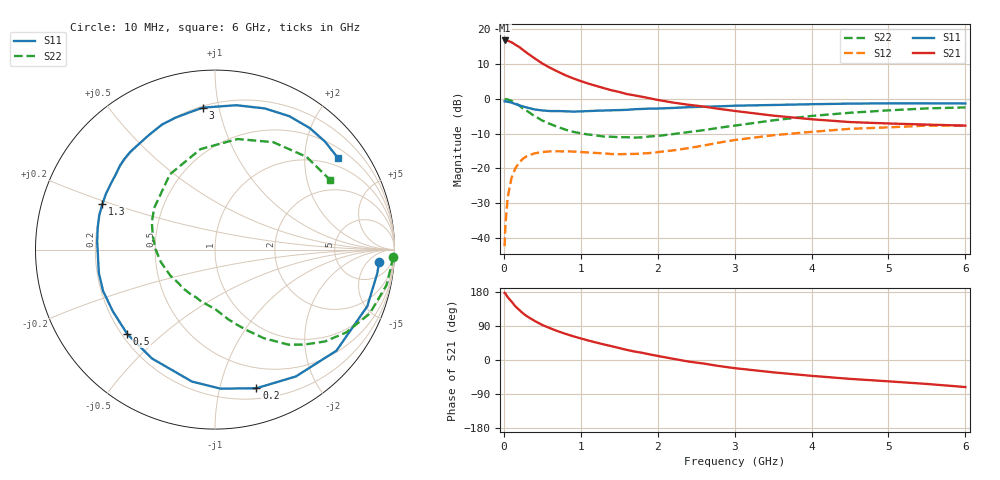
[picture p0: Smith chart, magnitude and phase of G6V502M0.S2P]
! SIEMENS Small Signal Semiconductors
! BFG193
! Si NPN RF Bipolar Junction Transistor in SOT223
! VCE = 0.5 V  IC = 2 mA
! Common Emitter S-Parameters:  August  1996
# GHz  S  MA  R  50
!  f  S11  S21  S12  S22
! GHz  MAG  ANG  MAG  ANG  MAG  ANG  MAG  ANG
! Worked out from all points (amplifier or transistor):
!   36 points, 10 MHz to 6 GHz, reference 50 ohm
!   highest |S21| = 16.8 dB at 10 MHz (marker M1)
!   |S21| within 3 dB of that: start of sweep to 265.8 MHz
!   unconditionally stable (mu >= 1): 1.313 GHz to end of sweep
!   at 250 MHz: K = 0.20, MSG = 15.6 dB, |S12| = -17.2 dB
!   at 1.4 GHz: K = 1.07, MAG = 7.5 dB, |S12| = -15.9 dB
!   at 6 GHz: K = 1.04, MAG = -1.2 dB, |S12| = -7.7 dB
!   S11 on the Smith chart (normalised r, x): 10 MHz: 13, -11; 200 MHz: 0.29, -1.30; 500 MHz: 0.22, -0.39; 1.3 GHz: 0.20, +0.19; 3 GHz: 0.21, +0.90; 6 GHz: 0.75, +2.84
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0.01  0.9175 -4.2  6.882 177.1  0.0076 88.4  0.9938 -2.4
0.02  0.9136 -8.4  6.88 175.4  0.0151 88.6  0.9874 -4.7
0.05  0.9055 -20.4  6.823 165.8  0.0381 78.0  0.976 -11.7
0.1  0.8803 -39.8  6.481 154.3  0.0727 68.4  0.9325 -22.5
0.15  0.8382 -57.5  5.98 141.6  0.1001 57.3  0.8652 -32.2
0.2  0.806 -73.4  5.537 132.2  0.1215 49.7  0.7981 -39.9
0.25  0.7755 -87.7  5.025 123.0  0.1377 42.4  0.7243 -47.0
0.3  0.7464 -99.9  4.557 115.5  0.15 36.8  0.6683 -52.4
0.4  0.7009 -120.1  3.812 103.2  0.1642 28.2  0.5627 -61.2
0.5  0.6784 -136.1  3.211 92.5  0.1712 21.1  0.4862 -68.1
0.6  0.665 -148.9  2.789 83.9  0.1751 16.5  0.4343 -73.9
0.7  0.6649 -159.7  2.457 76.1  0.1758 12.9  0.3941 -79.4
0.9  0.6532 -176.9  1.966 62.8  0.1741 7.8  0.3345 -89.2
1.1  0.6645 169.6  1.649 51.4  0.1687 5.1  0.3059 -100.4
1.3  0.677 157.9  1.42 41.1  0.1641 4.0  0.2861 -111.4
1.7  0.7066 138.5  1.117 22.3  0.1608 7.0  0.2761 -136.9
2.2  0.7369 120.0  0.881 3.3  0.1809 10.5  0.3102 -167.4
3  0.7938 94.9  0.668 -21.5  0.2552 6.4  0.4104 145.8
3.5  0.8131 81.6  0.572 -32.5  0.299 -4.4  0.489 120.9
4.5  0.8508 60.9  0.462 -49.8  0.3693 -24.2  0.6286 78.5
5.5  0.8589 44.5  0.425 -63.2  0.4111 -47.9  0.7262 45.4
6  0.8545 36.6  0.411 -71.4  0.4101 -61.1  0.7503 31.0
